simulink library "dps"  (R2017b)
settings: Solver=VariableStepAuto  StartTime=0.0  StopTime=10.0  RelTol=1e-3
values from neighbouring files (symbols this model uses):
  w = [196;186;150;145;140;105;85;83;85;80;80]    [readW.m]
undefined symbols (not defined in the file or in its folder): deadbeat, e, H, M, Manual, surf, T, z

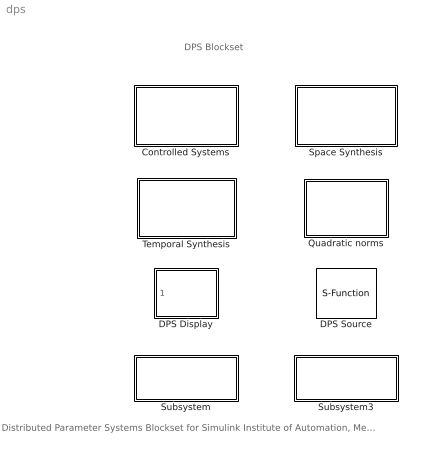
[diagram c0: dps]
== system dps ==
  note: Distributed Parameter Systems Blockset for Simulink Institute of Automation, Measurement and Applied Informatics, Mechanical Engineering Faculty Slovak University of Technology in Bratislava 2004 - 2018 For contact: gabriel.hulko@stuba.sk
  note: DPS Blockset
  Controlled Systems : Subsystem
      mask init:
      | [ix1,iy1,ic1,ix2,iy2,ix3,iy3,ix4,iy4,ixs1,iys1,ixs2,iys2,ixs3,iys3,ixb1,iyb1,ixb2,iyb2] = dpsh_ssr('icon');
  DPS Display : Subsystem  mask(Display){graphType=surf, pointCoord=M, elementsVar=e, showColor=on, minC=0, maxC=100, showDeform=off, deform=z, deformScale=0.001, showScope=off, responseVar=H, saveAvi=off, aviparam=0}
      mask prompts: graphType "Display type"; pointCoord "Nodal matrix"; elementsVar "Element matrix"; showColor "Show color"; minC "Min."; maxC "Max."; showDeform "Deformed shape"; deform "Deformation direction"; deformScale "Deformation factor"; showScope "Plot max-gain locations"; responseVar "Step-change responses"; saveAvi "Save animation to file"; aviparam "AVI parameters"
      mask help: Block displays spatio-temporal (distributed) variables on the definition domain and the time courses in the max-gain locations, each corresponding to the individual step-change response {H}i=1, n where n = total number of individual step-change responses.
      mask init:
      | [ix1,iy1,ic1,ix2,iy2,ix3,iy3,ix4,iy4,ix5,iy5,ic5,ixsin,iysin] = dpsh_display('icon');
  DPS Source : S-Function  FunctionName=sfun_input  Parameters='geom', struct('M',pointsCoord,'e',elementsVar), 'H', responseVar, 'quantity', equation, 'samplePeriod', samplePeriod, 'input', showInput  SFunctionDeploymentMode=off  EnableBusSupport=off  mask(Source){equation=w, responseVar=0, showInput=on, pointsCoord=M, elementsVar=e, samplePeriod=T}
      mask prompts: equation "Value"; responseVar "Response Var"; showInput "Display"; pointsCoord "Nodal matrix"; elementsVar "Element matrix"; samplePeriod "Sampling period"
      mask help: Block outputs and displays spatio-temporal (distributed) variables such as distributed reference W(x, k) or distributed disturbance D(x, k) on the definition domain. If the variable should not be displayed then uncheck Display option or simply use any of the signal sources blocks from Simulink library. The variable is displayed on the surface mesh defined by nodal and element matrices. The value of variable (Value parameter) addresses every node. In the case of constant and homogeneous variable it can be defined as "const * ones(NNOD, 1)". In the case of triangular surface elements defined by 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
      mask init:
      | [ix1,iy1,ic1,ix2,iy2,ix3,iy3,ix4,iy4,ix5,iy5,ic5,ixsin,iysin] = dpsh_input('icon');
  Quadratic norms : Subsystem
  Space Synthesis : Subsystem
      mask init:
      | [ix1,iy1,ic1,ix2,iy2,ix3,iy3,ix4,iy4,ixs1,iys1,ixs2,iys2,ixs3,iys3,ixb1,iyb1,ixb2,iyb2]=dpsh_ss('icon');
  Subsystem : Subsystem
  Subsystem3 : Subsystem
  Temporal Synthesis : Subsystem
      mask init:
      | [ix1,iy1,ic1,ix2,iy2,ixvs1,ixvs2,ixvs3,iyvs1,iyvs2,iyvs3,ixvb1,ixvb2,iyvb1,iyvb2,ixs1,iys1,ixs2,iys2,ixs3,iys3,ixb1,iyb1,ixb2,iyb2]=dpsh_pidcontrol('icon');

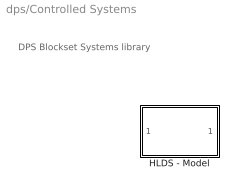
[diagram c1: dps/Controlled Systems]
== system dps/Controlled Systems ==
  note: DPS Blockset Systems library
  HLDS - Model : Subsystem  mask(System){StepResponse=H, samplePeriod=T, u_step=1}
      mask prompts: StepResponse "Responses to step changes"; samplePeriod "Sampling period"; u_step "Amplitudes of step changes"
      mask help: HLDS - Lumped-input / Distributed-output System with zero-order Hold units. Block computes the transient response of dynamic system Y(x, k) by summation on signal convolutions of distributed impulse functions {G(x, k)}i=1,n with their respective signal inputs {U(k)}i=1,n where n = total number of step-change responses in summation. Sampling period is assumed to be constant for all responses. Enter the step-change responses parameter as cell array of size (1,n). Each step-change response {H}i=1,n is stored in the individual cell of the cell array. The time samples of individual responses are st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
      mask init:
      | [ix1,iy1,ic1,ix2,iy2,ix3,iy3,ix4,iy4,ixs1,iys1,ixs2,iys2,ixs3,iys3,ixb1,iyb1,ixb2,iyb2] = dpsh_ssr('icon');

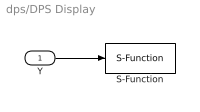
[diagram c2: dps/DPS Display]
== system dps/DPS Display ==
  Y : Inport
  S-Function : S-Function  FunctionName=sfun_display  Parameters='geom',struct('M',pointCoord,'e',elementsVar),'H',responseVar,'showScope',showScope,'cminmax',[minC maxC],'saveAvi',saveAvi,'aviparam',aviparam,'graphType',graphType,'showDeform',showDeform,'deform',deform,'deformKoeficient',deformScale  SFunctionDeploymentMode=off  EnableBusSupport=off
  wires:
  Y/1 -> S-Function/1

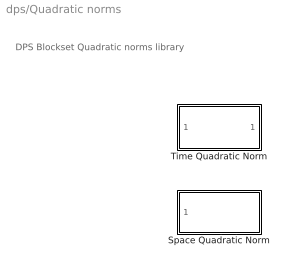
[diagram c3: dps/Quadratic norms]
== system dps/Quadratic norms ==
  note: DPS Blockset Quadratic norms library
  Space Quadratic Norm : Subsystem  mask(Quadratic Norm){StepResponse=H, showNorm=on}
      mask prompts: StepResponse "Responses to step changes"; showNorm "Show norm ||E||"
      mask help: This block computes the Quadratic norm of the input signal.
  Time Quadratic Norm : Subsystem  mask(Quadratic Norm){}
      mask help: This block computes the Quadratic norm of the input signal.

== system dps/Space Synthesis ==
  note: DPS Blockset Space synthesis library
  Space Synthesis : S-Function  FunctionName=sfun_ss  Parameters=PCH,weights  SFunctionDeploymentMode=off  EnableBusSupport=off  mask(Space Synthesis){PCH=H, weights=[]}
      mask prompts: PCH "Responses to step changes"; weights "Weighting coefficients"
      mask init:
      | [ix1,iy1,ic1,ix2,iy2,ix3,iy3,ix4,iy4,ixs1,iys1,ixs2,iys2,ixs3,iys3,ixb1,iyb1,ixb2,iyb2]=dpsh_ss('icon');

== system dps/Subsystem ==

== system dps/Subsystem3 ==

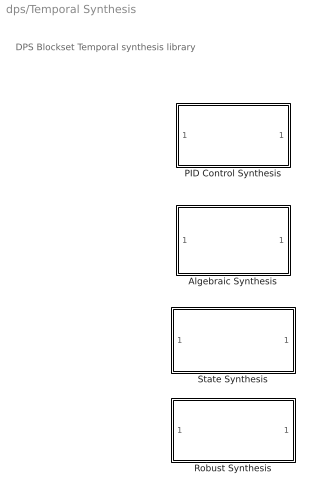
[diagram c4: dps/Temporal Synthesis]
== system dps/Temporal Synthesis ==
  note: DPS Blockset Temporal synthesis library
  Algebraic Synthesis : Subsystem  mask{kriterium=deadbeat, b=[], a=[], samplePeriod=T}
      mask prompts: kriterium "Method"; b "Numerators"; a "Denominators"; samplePeriod "Sampling period"
      mask init:
      | [ix1,iy1,ic1,ix2,iy2,ixvs1,ixvs2,ixvs3,iyvs1,iyvs2,iyvs3,ixvb1,ixvb2,iyvb1,iyvb2,ixs1,iys1,ixs2,iys2,ixs3,iys3,ixb1,iyb1,ixb2,iyb2]=dpsh_pidcontrol('icon');
  PID Control Synthesis : Subsystem  mask{method=Manual, r0=[], ri=[], rd=[], b=[], a=[], tau=[], StepResponse=H, weights=[], samplePeriod=T}
      mask prompts: method "PID parameters determination"; r0 "Proportional term (P)"; ri "Integral term (I)"; rd "Derivative term (D)"; b "Numerators"; a "Denominators"; StepResponse "Responses to step changes"; weights "Space weighting coefficients"; samplePeriod "Sampling period"
      mask init:
      | [ix1,iy1,ic1,ix2,iy2,ixvs1,ixvs2,ixvs3,iyvs1,iyvs2,iyvs3,ixvb1,ixvb2,iyvb1,iyvb2,ixs1,iys1,ixs2,iys2,ixs3,iys3,ixb1,iyb1,ixb2,iyb2]=dpsh_pidcontrol('icon');
  Robust Synthesis : Subsystem  mask{b=[], a=[], alfa=[], SamplePeriod=T}
      mask prompts: b "Numerators"; a "Denominators"; alfa "Filter parameters (alpha)"; SamplePeriod "Sampling period"
      mask init:
      | [ix1,iy1,ic1,ix2,iy2,ixvs1,ixvs2,ixvs3,iyvs1,iyvs2,iyvs3,ixvb1,ixvb2,iyvb1,iyvb2,ixs1,iys1,ixs2,iys2,ixs3,iys3,ixb1,iyb1,ixb2,iyb2]=dpsh_pidcontrol('icon');
  State Synthesis : Subsystem  mask{b=[], a=[], Q=[], R=[], SamplePeriod=T}
      mask prompts: b "Numerators"; a "Denominators"; Q "State weighting matrix (Q)"; R "Input weighting matrix (R)"; SamplePeriod "Sampling period"
      mask init:
      | [ix1,iy1,ic1,ix2,iy2,ixvs1,ixvs2,ixvs3,iyvs1,iyvs2,iyvs3,ixvb1,ixvb2,iyvb1,iyvb2,ixs1,iys1,ixs2,iys2,ixs3,iys3,ixb1,iyb1,ixb2,iyb2]=dpsh_pidcontrol('icon');

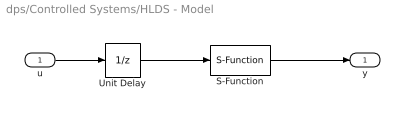
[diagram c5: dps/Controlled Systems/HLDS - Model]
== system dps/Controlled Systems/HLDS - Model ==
  u : Inport
  S-Function : S-Function  FunctionName=sfun_ssr  Parameters=samplePeriod, StepResponse, u_step  SFunctionDeploymentMode=off  EnableBusSupport=off
  Unit Delay : UnitDelay  SampleTime=-1
  y : Outport
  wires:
  S-Function/1 -> y/1
  u/1 -> Unit Delay/1
  Unit Delay/1 -> S-Function/1

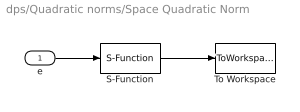
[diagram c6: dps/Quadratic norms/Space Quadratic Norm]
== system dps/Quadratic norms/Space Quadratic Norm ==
  e : Inport
  S-Function : S-Function  FunctionName=sfun_norm  Parameters=StepResponse,showNorm  SFunctionDeploymentMode=off  EnableBusSupport=off
  To Workspace : ToWorkspace  VariableName=dps_norm  SaveFormat=Structure  SampleTime=-1
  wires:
  S-Function/1 -> To Workspace/1
  e/1 -> S-Function/1

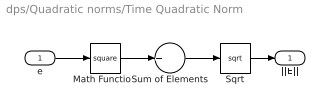
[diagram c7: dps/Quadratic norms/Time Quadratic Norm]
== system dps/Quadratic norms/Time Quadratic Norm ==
  e : Inport
  Math Function : Math  Operator=square
  Sqrt : Sqrt
  Sum of Elements : Sum  Inputs=+
  ||E|| : Outport
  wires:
  e/1 -> Math Function/1
  Math Function/1 -> Sum of Elements/1
  Sqrt/1 -> ||E||/1
  Sum of Elements/1 -> Sqrt/1

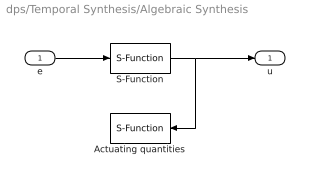
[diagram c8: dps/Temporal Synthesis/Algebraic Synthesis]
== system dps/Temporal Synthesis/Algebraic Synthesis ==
  e : Inport
  Actuating quantities : S-Function  FunctionName=sfun_scope  Parameters=length(H)  SFunctionDeploymentMode=off  EnableBusSupport=off
  S-Function : S-Function  FunctionName=sfun_algebra  Parameters=a,b,kriterium,samplePeriod  SFunctionDeploymentMode=off  EnableBusSupport=off
  u : Outport
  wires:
  S-Function/1 -> Actuating quantities/1, u/1
  e/1 -> S-Function/1

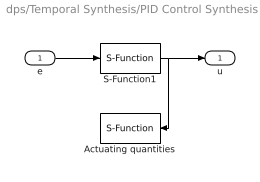
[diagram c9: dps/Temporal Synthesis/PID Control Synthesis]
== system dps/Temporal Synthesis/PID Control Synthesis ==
  e : Inport
  Actuating quantities : S-Function  FunctionName=sfun_scope  Parameters=length(H)  SFunctionDeploymentMode=off  EnableBusSupport=off
  S-Function1 : S-Function  FunctionName=sfun_psd  Parameters='method',method,'num',b,'den',a,'P',r0,'I',ri,'D',rd,'TAU',tau,'samplePeriod',samplePeriod,'weights',weights,'StepResponse',StepResponse  SFunctionDeploymentMode=off  EnableBusSupport=off
  u : Outport
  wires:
  S-Function1/1 -> Actuating quantities/1, u/1
  e/1 -> S-Function1/1

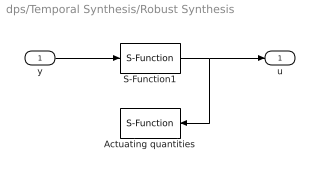
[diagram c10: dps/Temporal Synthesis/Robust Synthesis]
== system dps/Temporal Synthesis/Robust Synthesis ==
  y : Inport
  Actuating quantities : S-Function  FunctionName=sfun_scope  Parameters=length(H)  SFunctionDeploymentMode=off  EnableBusSupport=off
  S-Function1 : S-Function  FunctionName=sfun_robust  Parameters=a,b,alfa,SamplePeriod  SFunctionDeploymentMode=off  EnableBusSupport=off
  u : Outport
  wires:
  S-Function1/1 -> Actuating quantities/1, u/1
  y/1 -> S-Function1/1

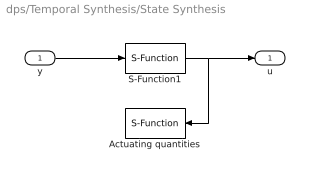
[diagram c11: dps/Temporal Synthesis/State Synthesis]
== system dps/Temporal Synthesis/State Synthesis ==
  y : Inport
  Actuating quantities : S-Function  FunctionName=sfun_scope  Parameters=length(H)  SFunctionDeploymentMode=off  EnableBusSupport=off
  S-Function1 : S-Function  FunctionName=sfun_state  Parameters=a,b,SamplePeriod,Q,R  SFunctionDeploymentMode=off  EnableBusSupport=off
  u : Outport
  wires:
  y/1 -> S-Function1/1
  S-Function1/1 -> Actuating quantities/1, u/1
